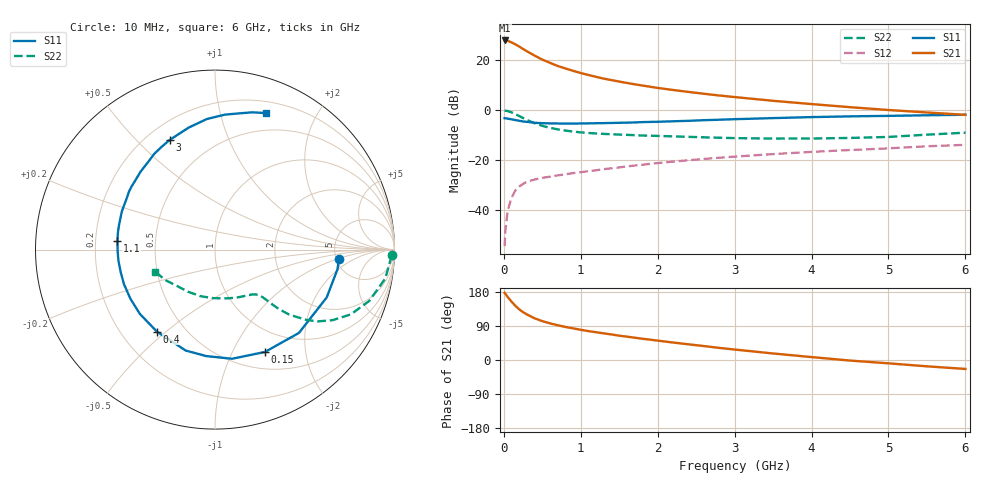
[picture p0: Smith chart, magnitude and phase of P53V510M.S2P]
! SIEMENS Small Signal Semiconductors
! BFP183
! Si NPN RF Bipolar Junction Transistor in SOT143
! VCE = 3.5 V  IC = 10 mA
! Common Emitter S-Parameters:  March  1996
# GHz  S  MA  R  50
!  f  S11  S21  S12  S22
! GHz  MAG  ANG  MAG  ANG  MAG  ANG  MAG  ANG
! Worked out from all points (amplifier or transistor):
!   36 points, 10 MHz to 6 GHz, reference 50 ohm
!   highest |S21| = 27.9 dB at 10 MHz (marker M1)
!   |S21| within 3 dB of that: start of sweep to 229 MHz
!   unconditionally stable (mu >= 1): 1.167 GHz to 5.537 GHz
!   at 250 MHz: K = 0.32, MSG = 27.0 dB, |S12| = -29.5 dB
!   at 1.4 GHz: K = 1.07, MAG = 16.0 dB, |S12| = -23.2 dB
!   at 6 GHz: K = 0.96, MSG = 6.0 dB, |S12| = -13.9 dB
!   lowest NFmin = 1.30 dB at 450 MHz
!   S11 on the Smith chart (normalised r, x): 10 MHz: 5.27, -1.10; 150 MHz: 0.71, -1.35; 400 MHz: 0.35, -0.47; 1.1 GHz: 0.29, +0.04; 3 GHz: 0.29, +0.63; 6 GHz: 0.31, +1.39
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0.01  0.6926 -4.5  24.93 177.3  0.0019 91.7  0.9853 -1.9
0.02  0.6912 -9.1  24.85 174.8  0.0039 84.3  0.9777 -3.9
0.05  0.677 -23.2  24.51 166.3  0.0098 81.6  0.9625 -9.6
0.1  0.659 -44.8  22.78 154.0  0.0177 69.6  0.906 -18.4
0.15  0.6345 -64.0  20.82 143.0  0.0249 62.2  0.8384 -25.5
0.2  0.6156 -81.1  18.85 133.7  0.0297 56.4  0.7637 -31.0
0.25  0.5953 -94.7  16.82 126.2  0.0334 51.5  0.6974 -35.0
0.3  0.5856 -106.2  15.14 120.3  0.0371 48.6  0.6393 -37.7
0.4  0.5599 -125.3  12.39 110.0  0.041 44.5  0.5499 -41.2
0.5  0.551 -139.4  10.32 102.6  0.0443 41.8  0.4872 -42.9
0.6  0.545 -149.8  8.892 96.7  0.0467 41.7  0.4442 -43.7
0.7  0.5425 -159.1  7.691 91.7  0.0496 41.0  0.4143 -44.1
0.9  0.5415 -173.5  6.153 83.5  0.0551 41.7  0.3742 -45.0
1.1  0.5457 174.9  5.079 76.2  0.0603 42.4  0.3501 -46.3
1.5  0.5608 157.7  3.743 64.2  0.0718 43.1  0.3254 -50.1
1.8  0.5783 145.9  3.124 56.1  0.0809 43.5  0.3115 -54.5
2.2  0.6005 133.7  2.543 46.1  0.0935 42.4  0.2995 -61.4
3  0.6615 112.3  1.835 27.6  0.1178 38.2  0.2766 -79.2
3.5  0.6956 102.1  1.544 17.2  0.1324 35.2  0.2707 -92.3
4.5  0.7537 85.9  1.151 -1.5  0.1596 27.8  0.2786 -122.5
5.5  0.7925 74.8  0.902 -16.7  0.1899 21.1  0.3242 -148.3
6  0.8113 69.7  0.809 -23.6  0.2029 16.7  0.3557 -159.8
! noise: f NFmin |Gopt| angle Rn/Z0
0.45  1.3  0.15  45  0.18
0.9  1.4  0.2  125  0.19
1.8  2.1  0.34  -170  0.14
